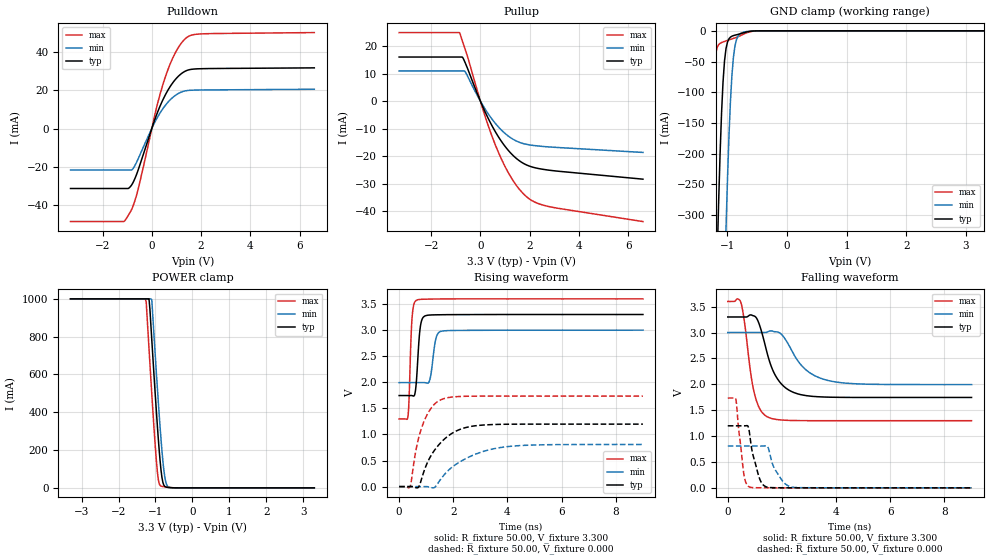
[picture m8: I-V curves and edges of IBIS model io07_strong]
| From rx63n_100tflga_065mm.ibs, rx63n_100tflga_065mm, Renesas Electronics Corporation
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[Model]   io07_strong
Model_type   I/O
Polarity   Non-Inverting
Enable   Active-High
Vinl  =   0.660V
Vinh  =   2.640V
Vmeas =   1.650V
Cref  =   30.00pF
| variable   typ   min   max
C_comp   3.960pF   3.960pF   3.960pF
| variable   typ   min   max
[Temperature Range]   45.000   105.000   -40.000
| variable   typ   min   max
[Voltage Range]   3.300V   3.000V   3.600V
| variable   typ   min   max
[Pullup Reference]   3.300V   3.000V   3.600V
| variable   typ   min   max
[Pulldown Reference]   0.000V   0.000V   0.000V
| variable   typ   min   max
[POWER Clamp Reference] 3.300V   3.000V   3.600V
| variable   typ   min   max
[GND Clamp Reference]   0.000V   0.000V   0.000V
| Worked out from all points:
|   slope of the pulldown table from 0 to 0.495 V, typ, clamps not added: 30.7 ohm
|   slope of the pullup table from 0 to 0.495 V, typ, clamps not added: 52.9 ohm
|   GND clamp passes 1 mA (typ) near -0.63 V on its own axis
|   POWER clamp passes 1 mA (typ) near -0.58 V on its own axis
|   rising waveform, R_fixture 50.00, V_fixture 3.300: 20-80 % time 122ps typ, 154ps min, 93.6ps max; typ from 1.75 V to 3.3 V
|   rising waveform, R_fixture 50.00, V_fixture 0.000: 20-80 % time 897ps typ, 1.38ns min, 529ps max; typ from 0 V to 1.2 V
|   falling waveform, R_fixture 50.00, V_fixture 3.300: 20-80 % time 638ps typ, 903ps min, 383ps max; typ from 3.3 V to 1.75 V
|   falling waveform, R_fixture 50.00, V_fixture 0.000: 20-80 % time 308ps typ, 424ps min, 213ps max; typ from 1.2 V to 0 V
[Pulldown]
| io07_strong Pulldown rx631_rx63n
| Thu Mar 22 17:15:49 2012
| voltage   I(typ)   I(min)   I(max)
-3.3V     -31.31mA   -21.63mA   -48.57mA
-1.15V    -31.31mA   -21.63mA   -48.57mA
-1.025V   -31.31mA   -21.63mA   -46.81mA
-800mV    -29.1mA    -21.49mA   -41.71mA
-600mV    -23.34mA   -17.13mA   -33.95mA
175mV     6.49mA     4.538mA    9.911mA
525mV     16.92mA    11.68mA    25.93mA
950mV     25.49mA    17.23mA    39.38mA
1.4V      30.18mA    19.75mA    47.31mA
1.7V      31.04mA    20.05mA    49.02mA
2.1V      31.26mA    20.14mA    49.45mA
6.6V      31.67mA    20.5mA     50.09mA
[Pullup]
| io07_strong Pullup rx631_rx63n
| Thu Mar 22 17:15:49 2012
| voltage   I(typ)   I(min)   I(max)
-3.3V     16.04mA    10.98mA    24.94mA
-850mV    16.04mA    10.98mA    24.94mA
-725mV    15.94mA    10.98mA    21.66mA
-625mV    14.1mA     10.75mA    19.05mA
175mV     -3.59mA    -2.649mA   -5.083mA
700mV     -12.53mA   -9.072mA   -17.96mA
1V        -16.45mA   -11.75mA   -23.79mA
1.325V    -19.76mA   -13.87mA   -28.89mA
1.95V     -23.51mA   -15.85mA   -35.33mA
2.3V      -24.41mA   -16.28mA   -37.1mA
2.9V      -25.25mA   -16.74mA   -38.59mA
6.6V      -28.4mA    -18.67mA   -43.82mA
[GND Clamp]
| io07_strong GNDClamp rx631_rx63n
| Thu Mar 22 17:15:49 2012
| voltage   I(typ)   I(min)   I(max)
-3.3V     -1A        -1A        -1A
-1.325V   -1A        -1A        -369.2mA
-1.3V     -928.6mA   -1A        -269.7mA
-1.25V    -694.8mA   -1A        -112.6mA
-1.175V   -376mA     -953.3mA   -27.44mA
-1.15V    -283.8mA   -837.7mA   -22.69mA
-1.075V   -83.42mA   -512.2mA   -18.16mA
-1.025V   -28.94mA   -323mA     -16.39mA
-925mV    -8.707mA   -71.38mA   -13.1mA
-850mV    -6.468mA   -14.65mA   -10.64mA
-675mV    -1.81mA    -1.082mA   -3.186mA
3.3V      0A         0A         0A
[POWER Clamp]
| io07_strong PWRClamp rx631_rx63n
| Thu Mar 22 17:15:49 2012
| voltage   I(typ)   I(min)   I(max)
-3.3V     1A         1A         1A
-1.275V   1A         1A         1A
-1.25V    1A         1A         982.1mA
-1.175V   1A         1A         736.6mA
-1.1V     784.3mA    995.9mA    498mA
-1V       476.2mA    683.1mA    204.7mA
-950mV    332.1mA    533mA      87.52mA
-875mV    143.3mA    321.7mA    12.76mA
-825mV    55.42mA    197.2mA    7.873mA
-750mV    8.12mA     59.94mA    5.513mA
-625mV    1.619mA    2.607mA    2.132mA
3.3V      0A         0A         0A
[Ramp]
dV/dt_r   0.719/896.57p  0.485/1.38n   1.041/529.77p
dV/dt_f   0.933/636.94p  0.604/902.43p  1.382/382.70p
R_load = 50.00ohm
[Rising Waveform]
| io07_strong Rising-High rx631_rx63n
| Thu Mar 22 17:15:49 2012
R_fixture = 50.00
V_fixture = 3.300
V_fixture_min = 3.000
V_fixture_max = 3.600
C_fixture = 0.00pF
| Time   V(typ)   V(min)   V(max)
0s        1.746V     1.994V     1.297V
325ps     1.746V     1.994V     1.341V
480ps     1.744V     1.994V     3.254V
645ps     2.076V     1.994V     3.575V
785ps     3.073V     1.994V     3.59V
995ps     3.28V      1.989V     3.594V
1.135ns   3.29V      2.053V     3.596V
1.345ns   3.294V     2.811V     3.597V
1.52ns    3.295V     2.974V     3.598V
9ns       3.3V       3V         3.6V
[Rising Waveform]
| io07_strong Rising-Low rx631_rx63n
| Thu Mar 22 17:15:49 2012
R_fixture = 50.00
V_fixture = 0.000
C_fixture = 0.00pF
| Time   V(typ)   V(min)   V(max)
0s        0V         0V         0V
405ps     0V         0V         1mV
595ps     -16mV      0V         626mV
705ps     -17mV      0V         901mV
875ps     227mV      0V         1.192V
1.295ns   689mV      -20mV      1.575V
1.63ns    892mV      206mV      1.683V
2.375ns   1.12V      513mV      1.731V
3.68ns    1.193V     744mV      1.735V
9ns       1.198V     808mV      1.735V
[Falling Waveform]
| io07_strong Falling-High rx631_rx63n
| Thu Mar 22 17:15:49 2012
R_fixture = 50.00
V_fixture = 3.300
V_fixture_min = 3.000
V_fixture_max = 3.600
C_fixture = 0.00pF
| Time   V(typ)   V(min)   V(max)
0s        3.3V       3V         3.6V
475ps     3.3V       3V         3.592V
970ps     3.32V      3V         1.852V
1.175ns   3.14V      3V         1.533V
1.48ns    2.552V     3.014V     1.367V
1.775ns   2.155V     3.014V     1.323V
2.19ns    1.91V      2.815V     1.304V
2.82ns    1.788V     2.311V     1.298V
3.705ns   1.752V     2.073V     1.297V
9ns       1.746V     1.994V     1.297V
[Falling Waveform]
| io07_strong Falling-Low rx631_rx63n
| Thu Mar 22 17:15:49 2012
R_fixture = 50.00
V_fixture = 0.000
C_fixture = 0.00pF
| Time   V(typ)   V(min)   V(max)
0s        1.198V     808mV      1.735V
295ps     1.198V     808mV      1.718V
600ps     1.198V     808mV      245mV
810ps     1.031V     808mV      14mV
915ps     671mV      808mV      5mV
1.155ns   208mV      808mV      2mV
1.465ns   12mV       799mV      1mV
1.755ns   3mV        346mV      0V
2.365ns   1mV        15mV       0V
9ns       0V         0V         0V
